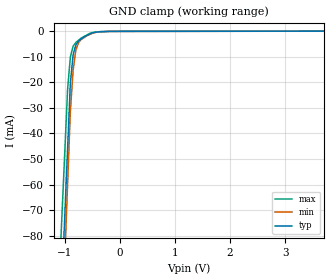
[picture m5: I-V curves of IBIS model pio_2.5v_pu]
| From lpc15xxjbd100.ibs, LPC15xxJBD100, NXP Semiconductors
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[Model] pio_2.5v_pu
Model_type Input
Vinl = 750.000mV
Vinh = 1.75000V
C_comp 598.000fF 598.000fF 598.000fF
| variable typ   min   max
[Voltage Range] 2.50000V 2.25000V 2.75000V
[POWER Clamp Reference] 2.50000V 2.25000V 2.75000V
[GND Clamp Reference] 0.00000V 0.00000V 0.00000V
[Temperature Range]   25   85   -40
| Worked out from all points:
|   GND clamp passes 1 mA (typ) near -0.53 V on its own axis
[GND Clamp]
-2.5V     -843.4mA   -940.4mA   -768.4mA
-950mV    -45.95mA   -59.81mA   -22.75mA
-900mV    -20.22mA   -31.4mA    -10.11mA
-850mV    -9.279mA   -15.24mA   -5.874mA
-800mV    -5.352mA   -7.376mA   -4.407mA
-750mV    -3.857mA   -4.408mA   -3.532mA
-700mV    -2.939mA   -3.178mA   -2.657mA
-550mV    -1.166mA   -1.284mA   -892.5uA
-400mV    -269.3uA   -271.4uA   -246.2uA
-200mV    -94.1uA    -81.77uA   -80.66uA
5V        31.77uA    45.17uA    23.92uA
[POWER Clamp]
-2.5V     0A         0A         0A
5V        0A         0A         0A
